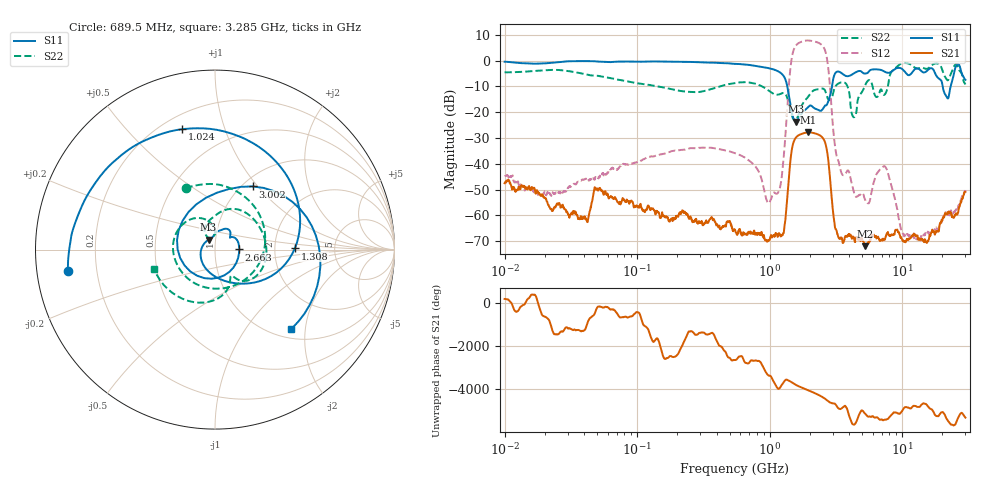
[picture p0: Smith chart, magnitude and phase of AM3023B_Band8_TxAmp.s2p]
# Hz S DB R 50.0
!freq dBS11 angS11 dBS21 angS21 dBS12 angS12 dBS22 angS22
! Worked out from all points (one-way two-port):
!   1601 points, 10 MHz to 30 GHz, reference 50 ohm
!   highest |S21| = -27.78 dB at 1.952 GHz (marker M1); lowest = -71.9 dB at 5.232 GHz (marker M2)
!   lowest |S11| = -23.6 dB at 1.574 GHz (marker M3), VSWR 1.14, Z = 46.2 + j5.11 ohm
!   |S11| at or under -10 dB: 1.358 GHz to 2.957 GHz (1.598 GHz wide, 74.1 % of centre); 20.23 GHz to 23.23 GHz (3.001 GHz wide, 13.8 % of centre)
!   |S22| runs from -23.2 to -0.9 dB; largest |S21 - S12| = 2.5
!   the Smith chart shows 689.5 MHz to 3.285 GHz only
!   S11 on the Smith chart (normalised r, x): 689.5 MHz: 0.09, -0.07; 1.024 GHz: 0.28, +0.72; 1.308 GHz: 2.60, +0.04; 2.663 GHz: 1.31, +0.00; 3.002 GHz: 1.11, +0.94; 3.285 GHz: 1.18, -1.68
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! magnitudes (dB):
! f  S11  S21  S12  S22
! 10 MHz  -0.4  -47.5  -44.8  -4.6
! 38.04 MHz  -0.2  -61.4  -46.4  -5.0
! 49.59 MHz  -0.4  -49.6  -45.1  -5.9
! 144.7 MHz  -0.4  -58.9  -36.6  -10.0
! 547.7 MHz  -1.3  -65.5  -35.9  -8.7
! 689.5 MHz  -1.6  -66.6  -38.5  -8.5
! 1.024 GHz  -3.2  -67.6  -53.8  -12.3
! 1.19 GHz  -4.5  -67.3  -49.6  -13.0
! 1.308 GHz  -7.0  -62.4  -30.6  -12.8
! 1.439 GHz  -17.5  -38.1  -2.4  -19.4
! 1.574 GHz  -23.6  -29.9  5.7  -23.1
! 1.952 GHz  -18.0  -27.8  7.8  -14.0
! 2.084 GHz  -17.7  -27.9  7.6  -12.1
! 2.663 GHz  -17.4  -33.0  2.7  -12.6
! 3.002 GHz  -7.8  -58.0  -25.5  -13.0
! 3.285 GHz  -4.2  -68.2  -38.6  -9.0
! 4.326 GHz  -4.9  -68.5  -51.0  -22.0
! 5.232 GHz  -5.0  -71.9  -53.7  -9.8
! 7.926 GHz  -4.8  -67.7  -44.9  -7.9
! 10.03 GHz  -3.3  -69.5  -66.4  -1.1
! 13.2 GHz  -3.1  -69.3  -69.1  -3.1
! 30 GHz  -7.5  -50.8  -50.2  -9.3
